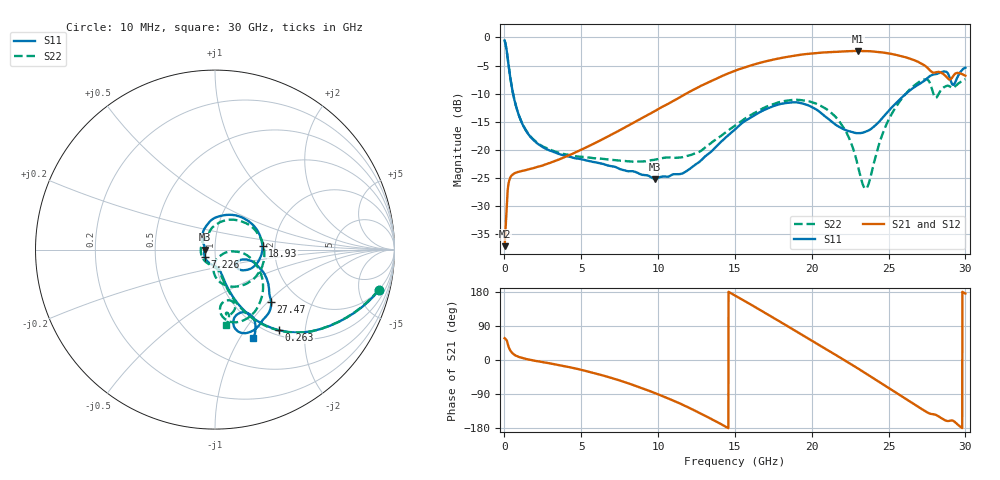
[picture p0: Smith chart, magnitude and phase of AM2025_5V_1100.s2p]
!Keysight Technologies,N5245B,MY58422270,A.16.20.02
!Date: Tuesday, July 14, 2026 01:09:47
!Correction: S11(C  2-Port  )
!S21(C  2-Port  )
!S12(C  2-Port  )
!S22(C  2-Port  )
!S2P File: Measurements: S11, S21, S12, S22:
# Hz S  dB  R 50
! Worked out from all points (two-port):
!   3201 points, 10 MHz to 30 GHz, reference 50 ohm
!   highest |S21| = -2.39 dB at 23.03 GHz (marker M1); lowest = -37.1 dB at 10 MHz (marker M2)
!   |S21| within 3 dB of the highest: 15.57 GHz to 27.53 GHz (11.96 GHz wide, 55.5 % of centre)
!   lowest |S11| = -25.1 dB at 9.766 GHz (marker M3), VSWR 1.12, Z = 44.8 - j0.0426 ohm
!   |S11| at or under -10 dB: 560.9 MHz to 26.13 GHz (25.57 GHz wide, 192 % of centre)
!   |S22| runs from -26.9 to -0.6 dB; largest |S21 - S12| = 0.0094
!   S11 on the Smith chart (normalised r, x): 10 MHz: 1.97, -7.69; 263 MHz: 1.09, -1.46; 7.226 GHz: 0.89, -0.07; 18.93 GHz: 1.72, +0.07; 27.47 GHz: 1.46, -1.05; 30 GHz: 0.82, -1.14
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1e7  -0.53 -13.9  -37.08 57.5  -36.01 93.5  -0.55 -13.8
2.630406e8  -4.81 -51.5  -26.01 35.5  -26.04 35.9  -4.84 -51.8
6.191719e8  -10.75 -68.8  -24.17 14.6  -24.17 14.6  -10.73 -69.6
1.612591e9  -17.40 -75.3  -23.40 1.0  -23.38 1.0  -17.33 -77.6
5.014581e9  -21.63 -109.7  -19.92 -26.1  -19.92 -26.1  -21.19 -120.4
7.226344e9  -23.02 -144.4  -16.89 -50.6  -16.89 -50.6  -21.80 -161.7
9.766122e9  -25.13 -179.5  -13.11 -86.7  -13.11 -86.7  -21.74 152.7
1.000979e10  -24.93 179.5  -12.73 -90.6  -12.72 -90.6  -21.60 148.0
1.270889e10  -22.05 148.4  -8.71 -139.8  -8.71 -139.9  -20.27 110.2
1.5005e10  -16.35 103.9  -5.92 170.2  -5.91 170.2  -15.67 74.6
1.677628e10  -13.05 58.9  -4.40 128.7  -4.39 128.6  -12.66 36.9
1.893182e10  -11.52 3.9  -3.21 77.0  -3.21 77.0  -11.07 -15.5
2.000958e10  -12.37 -21.1  -2.83 50.9  -2.83 50.8  -11.51 -41.2
2.185584e10  -16.00 -39.3  -2.51 6.2  -2.51 6.2  -15.15 -83.6
2.302732e10  -17.02 -31.9  -2.39 -22.9  -2.38 -22.9  -23.10 -91.1
2.360838e10  -16.64 -24.6  -2.43 -37.7  -2.42 -37.7  -26.63 -38.8
2.500479e10  -13.05 -17.9  -2.83 -73.8  -2.83 -73.9  -14.61 -10.7
2.644806e10  -9.28 -31.3  -3.82 -111.1  -3.83 -111.2  -9.06 -40.8
2.746959e10  -7.36 -43.1  -5.24 -137.1  -5.25 -137.2  -7.44 -71.2
2.807877e10  -6.52 -55.1  -6.20 -144.9  -6.19 -144.9  -10.73 -76.6
2.901595e10  -7.47 -76.0  -7.46 -160.0  -7.45 -160.1  -8.76 -80.2
3e10  -5.37 -66.9  -6.79 175.4  -6.74 175.4  -7.41 -82.0
